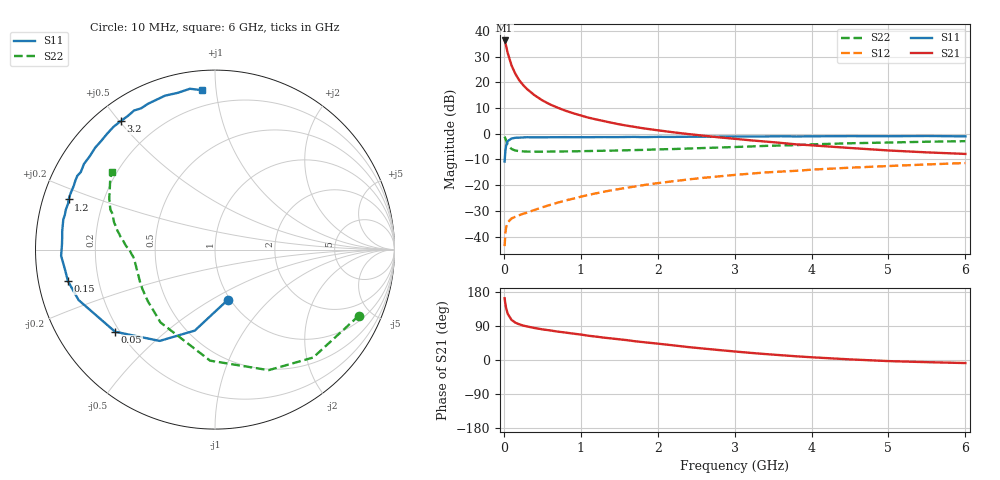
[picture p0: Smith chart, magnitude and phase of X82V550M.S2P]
! SIEMENS Small Signal Semiconductors
! BFP136W
! Si NPN RF Bipolar Junction Transistor in SOT343
! VCE = 2.5 V  IC = 50 mA
! Common Emitter S-Parameters:  September  1994
# GHz  S  MA  R  50
!  f  S11  S21  S12  S22
! GHz  MAG  ANG  MAG  ANG  MAG  ANG  MAG  ANG
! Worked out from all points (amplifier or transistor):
!   40 points, 10 MHz to 6 GHz, reference 50 ohm
!   highest |S21| = 36.3 dB at 10 MHz (marker M1)
!   |S21| within 3 dB of that: start of sweep to 35.92 MHz
!   unconditionally stable (mu >= 1): 635.7 MHz to 2.832 GHz
!   at 200 MHz: K = 0.55, MSG = 26.3 dB, |S12| = -31.7 dB
!   at 1.5 GHz: K = 1.12, MAG = 10.5 dB, |S12| = -21.5 dB
!   at 6 GHz: K = 0.97, MSG = 1.8 dB, |S12| = -11.4 dB
!   S11 on the Smith chart (normalised r, x): 10 MHz: 0.98, -0.59; 50 MHz: 0.18, -0.35; 150 MHz: 0.09, -0.11; 1.2 GHz: 0.08, +0.17; 3.2 GHz: 0.07, +0.50; 6 GHz: 0.11, +0.92
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0.01  0.2885 -75.6  65.64 163.0  0.0065 71.5  0.8825 -24.6
0.02  0.465 -104.0  58.29 148.0  0.0116 61.1  0.8129 -47.7
0.03  0.5948 -121.2  50.79 136.8  0.0151 51.4  0.7353 -66.0
0.05  0.7207 -140.6  37.62 122.0  0.0189 39.4  0.6195 -92.5
0.1  0.8103 -159.7  21.4 105.8  0.0225 32.0  0.5068 -126.8
0.15  0.8377 -167.8  14.67 98.5  0.0243 32.4  0.4717 -142.6
0.2  0.8426 -172.1  11.04 94.2  0.026 34.1  0.4603 -151.3
0.25  0.8505 -175.4  8.918 91.0  0.0278 36.4  0.4548 -156.9
0.3  0.8581 -177.7  7.459 88.6  0.0291 39.2  0.4508 -160.7
0.4  0.853 178.2  5.619 84.4  0.033 43.8  0.4495 -165.6
0.5  0.8541 175.5  4.484 80.9  0.0371 47.1  0.4499 -168.7
0.6  0.8575 173.2  3.737 78.1  0.0412 49.8  0.451 -170.7
0.7  0.8593 170.6  3.222 74.9  0.0457 52.6  0.4527 -172.1
0.9  0.8587 167.0  2.52 69.7  0.0546 55.2  0.456 -174.6
1.1  0.8577 162.5  2.061 64.0  0.0646 56.9  0.4619 -176.1
1.2  0.8622 161.1  1.904 61.7  0.0695 57.3  0.4655 -176.8
1.7  0.8703 151.8  1.364 49.6  0.0941 57.0  0.4826 179.5
2.2  0.8703 143.4  1.072 38.7  0.1192 54.5  0.5053 176.0
3.2  0.888 126.3  0.749 18.9  0.1674 46.2  0.5661 167.0
4.5  0.9017 108.0  0.53 1.6  0.2191 34.2  0.6545 154.2
5.5  0.907 98.9  0.435 -5.7  0.2533 26.2  0.7013 146.4
6  0.8913 94.6  0.406 -8.1  0.2701 21.8  0.7188 143.1
